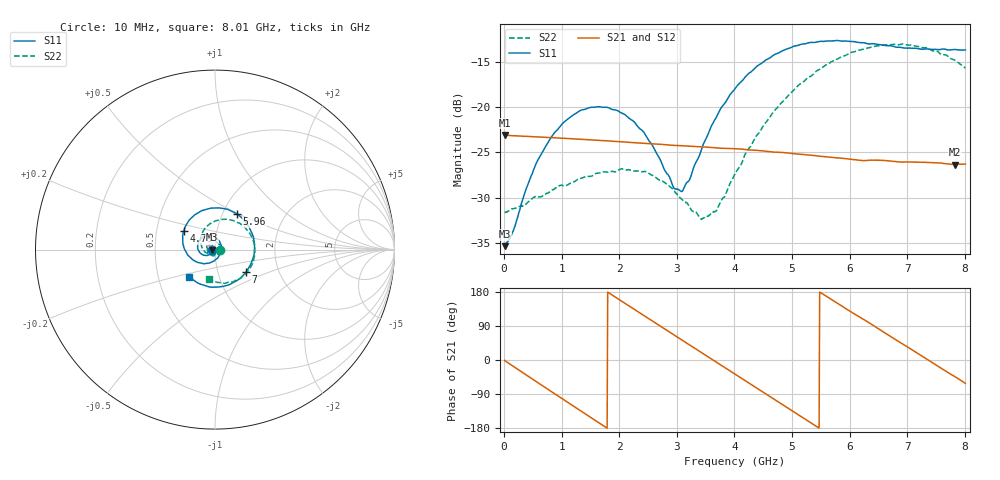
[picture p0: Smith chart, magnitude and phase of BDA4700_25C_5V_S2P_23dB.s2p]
!Agilent Technologies,E5071B,MY42404982,A.09.10
!Date: Mon Oct 20 13:37:59 2025
!Data & Calibration Information:
!Freq	S11:SOLT2(ON)	S21:SOLT2(ON)	S12:SOLT2(ON)	S22:SOLT2(ON)
# Hz S RI R 50
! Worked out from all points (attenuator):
!   801 points, 10 MHz to 8.01 GHz, reference 50 ohm
!   highest |S21| = -23.08 dB at 10 MHz (marker M1); lowest = -26.3 dB at 7.83 GHz (marker M2)
!   lowest |S11| = -35.4 dB at 10 MHz (marker M3), VSWR 1.03, Z = 48.3 - j0.103 ohm
!   |S11| at or under -10 dB: start of sweep to end of sweep
!   |S22| runs from -32.4 to -13.0 dB; largest |S21 - S12| = 0.00055
!   S11 on the Smith chart (normalised r, x): 10 MHz: 0.97, -0.00; 4.79 GHz: 0.69, +0.15; 5.96 GHz: 1.17, +0.49; 7 GHz: 1.37, -0.35; 8.01 GHz: 0.72, -0.23
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1e7  -0.017 -0.00107  0.0701 -0.0015  0.0701 -0.00155  0.0262 -0.000825
1.5e8  -0.018 -0.00944  0.067 -0.0187  0.067 -0.0187  0.0264 -0.00721
4.2e8  -0.028 -0.0254  0.0505 -0.047  0.0505 -0.047  0.02 -0.0222
7e8  -0.049 -0.0329  0.0221 -0.0646  0.0221 -0.0645  0.00582 -0.0323
1.03e9  -0.0791 -0.0223  -0.0165 -0.0653  -0.0165 -0.0653  -0.0167 -0.0327
1.35e9  -0.0965 0.00716  -0.0479 -0.0461  -0.048 -0.0461  -0.0365 -0.0176
2.09e9  -0.0485 0.0776  -0.0559 0.0317  -0.056 0.0317  -0.0288 0.0348
2.68e9  0.0236 0.048  -0.00273 0.0624  -0.00271 0.0624  0.0139 0.0373
2.95e9  0.0344 0.00941  0.0249 0.0563  0.025 0.0562  0.0261 0.0226
3.1e9  0.0314 -0.0141  0.0381 0.0479  0.038 0.048  0.0288 0.0105
3.41e9  0.00257 -0.056  0.0563 0.022  0.0564 0.022  0.0205 -0.0128
3.54e9  -0.0168 -0.0686  0.0594 0.00899  0.0595 0.00893  0.0127 -0.0215
3.7e9  -0.0469 -0.0767  0.0591 -0.00718  0.0592 -0.00732  -0.00121 -0.0272
4.01e9  -0.1087 -0.065  0.0469 -0.0356  0.0469 -0.0356  -0.0333 -0.0265
4.79e9  -0.1745 0.102  -0.0225 -0.0516  -0.0223 -0.0517  -0.0796 0.0664
5.35e9  -0.067 0.2189  -0.053 -0.0111  -0.053 -0.0114  -0.0155 0.1498
5.96e9  0.1233 0.1971  -0.0355 0.0377  -0.0356 0.0377  0.1239 0.1522
6.68e9  0.2187 -0.0195  0.0213 0.0457  0.0214 0.0457  0.2213 -0.00198
7e9  0.1742 -0.1225  0.0408 0.0285  0.0409 0.0283  0.2031 -0.0886
7.43e9  0.0469 -0.2039  0.0491 -0.00545  0.0491 -0.00555  0.1171 -0.1697
7.83e9  -0.0918 -0.1881  0.0346 -0.0336  0.0346 -0.0338  0.00995 -0.1819
8.01e9  -0.143 -0.1512  0.023 -0.0426  0.0231 -0.0427  -0.0335 -0.1616
